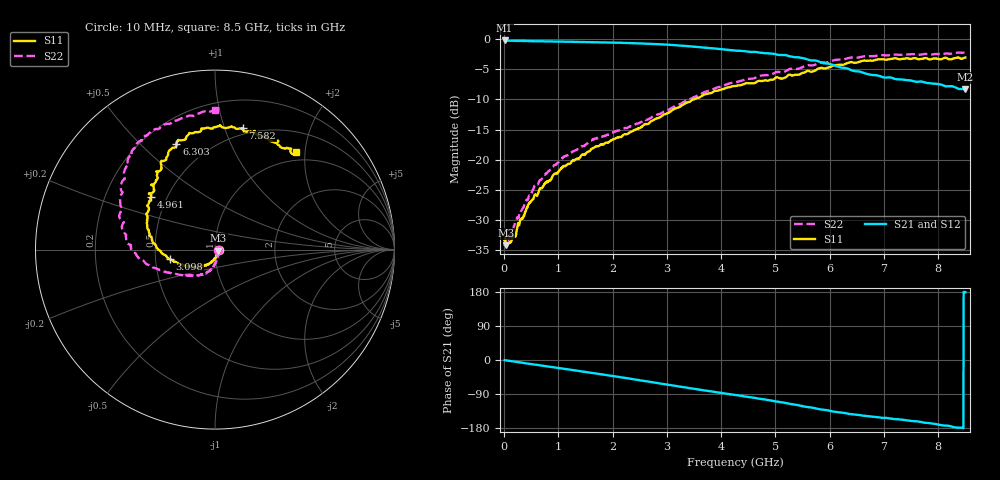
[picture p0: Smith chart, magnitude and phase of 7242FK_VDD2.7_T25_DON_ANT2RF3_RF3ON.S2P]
!Agilent Technologies,E5071C,MY46417908,A.11.23
!Date: Wed Dec 09 15:39:40 2020
!Data & Calibration Information:
!Freq	S11:SOLT2(ON)	S21:SOLT2(ON)	S12:SOLT2(ON)	S22:SOLT2(ON)
!PortZ  Port1:50+j0  Port2:50+j0
!Above PortZ is port z conversion or system Z0 setting when saving the data.
!When reading, reference impedance value at option line is always used.
# Hz S dB R 50
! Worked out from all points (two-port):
!   1601 points, 10 MHz to 8.5 GHz, reference 50 ohm
!   highest |S21| = -0.23 dB at 10 MHz (marker M1); lowest = -8.3 dB at 8.5 GHz (marker M2)
!   |S21| within 3 dB of the highest: start of sweep to 5.541 GHz
!   lowest |S11| = -34.2 dB at 36.53 MHz (marker M3), VSWR 1.04, Z = 51.9 - j0.547 ohm
!   |S11| at or under -10 dB: start of sweep to 3.486 GHz; 3.495747 GHz to 3.496637 GHz (890.1 kHz wide, 0.0255 % of centre)
!   |S22| runs from -34.3 to -2.2 dB; largest |S21 - S12| = 0.004
!   S11 on the Smith chart (normalised r, x): 10 MHz: 1.04, -0.00; 3.098 GHz: 0.60, -0.07; 4.961 GHz: 0.41, +0.31; 6.303 GHz: 0.33, +0.65; 7.582 GHz: 0.44, +1.16; 8.5 GHz: 0.85, +1.81
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1e7  -33.36 -1.7  -0.23 -0.3  -0.23 -0.4  -34.34 -9.9
3.653125e7  -34.19 -15.6  -0.26 -0.9  -0.26 -1.0  -33.81 -15.4
8.959375e7  -33.80 -29.9  -0.27 -2.0  -0.27 -2.1  -33.05 -29.1
1.798e8  -32.80 -49.0  -0.28 -4.0  -0.29 -4.0  -31.05 -48.0
4.398062e8  -27.54 -80.1  -0.32 -9.5  -0.32 -9.5  -26.65 -73.2
5.671562e8  -25.81 -90.6  -0.36 -12.1  -0.36 -12.1  -24.37 -82.9
1.081862e9  -21.26 -113.7  -0.43 -22.7  -0.43 -22.7  -19.73 -97.6
1.426769e9  -19.23 -124.7  -0.49 -30.0  -0.48 -30.1  -17.82 -106.7
1.66555e9  -17.95 -129.8  -0.52 -35.1  -0.53 -35.1  -16.53 -112.9
2.137806e9  -16.22 -139.9  -0.61 -45.3  -0.62 -45.3  -15.08 -125.8
2.843538e9  -13.08 -159.9  -0.84 -61.1  -0.85 -61.1  -12.46 -143.7
3.098238e9  -11.79 -168.0  -0.98 -66.9  -0.98 -67.0  -11.38 -150.2
3.70315e9  -9.18 173.9  -1.43 -80.4  -1.43 -80.4  -8.76 -165.1
4.255e9  -7.79 158.0  -1.89 -92.2  -1.89 -92.2  -7.13 -176.4
4.960731e9  -6.70 140.5  -2.42 -108.1  -2.40 -108.1  -5.72 168.5
5.671769e9  -5.41 124.0  -3.55 -125.6  -3.51 -125.6  -4.37 148.4
6.303212e9  -4.06 110.1  -4.82 -140.5  -4.84 -140.5  -3.27 135.2
6.621588e9  -3.56 102.5  -5.60 -147.1  -5.63 -146.9  -2.86 130.1
7.088538e9  -3.35 90.9  -6.35 -153.7  -6.38 -153.9  -2.70 123.9
7.582019e9  -3.16 77.1  -7.07 -161.7  -7.08 -161.5  -2.50 116.2
7.94815e9  -3.23 66.2  -7.40 -168.8  -7.43 -168.9  -2.47 107.9
8.5e9  -3.06 50.3  -8.35 179.0  -8.41 179.1  -2.19 90.1
